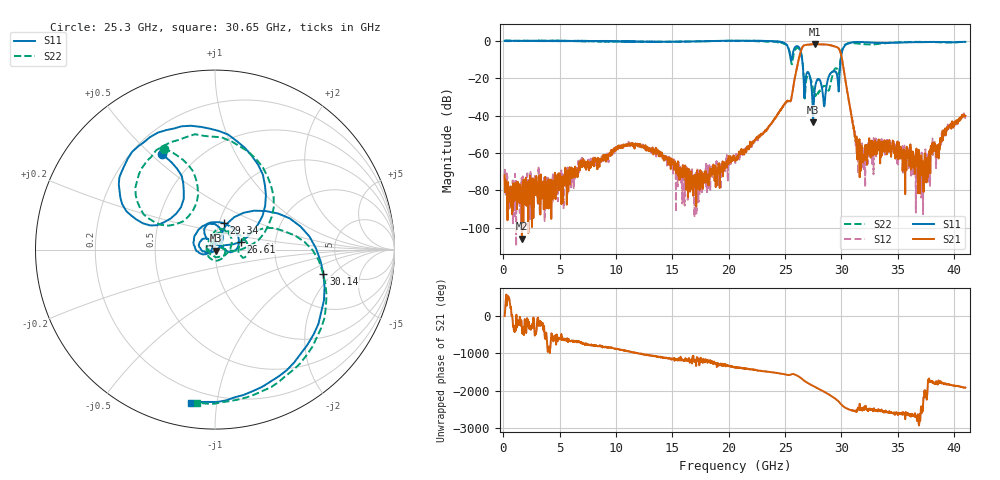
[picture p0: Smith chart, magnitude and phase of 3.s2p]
!The following data was pulled from an Agilent PNA
!This sNp file was generated from the data in the RF Test software
!NOTE:  Smoothing/Math/Corrections applied on any given trace ARE included in the data saved here
# MHz S dB R 50
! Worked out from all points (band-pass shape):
!   1601 points, 100 MHz to 41 GHz, reference 50 ohm
!   highest |S21| = -1.77 dB at 27.66 GHz (marker M1); lowest = -105.7 dB at 1.634 GHz (marker M2)
!   |S21| within 3 dB of the highest: 26.43 GHz to 29.83 GHz (3.397 GHz wide, 12.1 % of centre)
!   lowest |S11| = -43.6 dB at 27.48 GHz (marker M3), VSWR 1.01, Z = 50.4 - j0.533 ohm
!   |S11| at or under -10 dB: 25.49715 GHz to 25.57813 GHz (80.99 MHz wide, 0.317 % of centre); 26.51 GHz to 29.94 GHz (3.426 GHz wide, 12.1 % of centre)
!   |S22| runs from -30.9 to 0.2 dB; largest |S21 - S12| = 0.0062
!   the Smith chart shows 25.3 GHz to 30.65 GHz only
!   S11 on the Smith chart (normalised r, x): 25.3 GHz: 0.32, +0.54; 26.61 GHz: 1.33, +0.12; 29.34 GHz: 1.06, +0.32; 30.14 GHz: 3.52, -1.55; 30.65 GHz: 0.12, -0.85
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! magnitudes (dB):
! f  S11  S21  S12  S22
! 100 MHz  0.0  -71.9  -73.6  0.0
! 1.634 GHz  0.0  -105.7  -82.5  -0.1
! 6.925 GHz  -0.1  -64.1  -66.4  -0.2
! 13.75 GHz  -0.5  -59.1  -59.9  -0.5
! 16.95 GHz  -0.3  -72.6  -94.2  -0.3
! 20.55 GHz  0.1  -62.5  -63.3  -0.1
! 25.3 GHz  -4.3  -32.2  -32.1  -4.0
! 26.2 GHz  -3.3  -10.1  -10.1  -4.0
! 26.61 GHz  -16.5  -2.7  -2.7  -15.5
! 27.38 GHz  -27.4  -1.8  -1.8  -22.7
! 27.48 GHz  -43.6  -1.8  -1.8  -25.5
! 27.66 GHz  -24.8  -1.8  -1.8  -28.4
! 27.96 GHz  -20.6  -1.9  -1.8  -27.2
! 28.5 GHz  -34.4  -1.9  -2.0  -24.1
! 29.34 GHz  -16.2  -2.9  -2.9  -15.7
! 29.73 GHz  -25.7  -3.9  -3.9  -17.6
! 30.14 GHz  -4.2  -13.0  -13.0  -3.5
! 30.65 GHz  -1.3  -32.2  -32.2  -1.3
! 31.47 GHz  -0.6  -62.6  -60.3  -1.4
! 34.2 GHz  -1.1  -57.5  -57.9  -1.1
! 37.11 GHz  -0.7  -64.6  -59.7  -0.6
! 41 GHz  -0.5  -40.1  -39.6  -0.6
